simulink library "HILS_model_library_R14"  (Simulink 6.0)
undefined symbols (not defined in the file or in its folder): hilsmdl
libraries: simulink x47, simulink_extras x9, HILS_model_library x3
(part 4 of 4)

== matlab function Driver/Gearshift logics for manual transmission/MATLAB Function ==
function [indicator, skip_nr, req_gear, simtime_prev_out] = fGearVectoMisc(indicator_in, skip_nr_in, last_req_gear, simtime_prev, simtime, act_vehicle_speed, act_rotational_speed,...
                                                            act_gear, clutches_locked, acc_pedal, ref_drive_cycle, gbx, VectoMisc, VectoICE, VectoShiftUp, VectoShiftDown)

% VectoMisc(1,1)    ... dat.vecto.vehicle.mass.value
% VectoMisc(1,2)    ... dat.vecto.fg.ratio.value
% VectoMisc(1,3)    ... dat.vecto.fg.efficiency.value
% VectoMisc(1,4)    ... dat.vecto.wheel.radius.value
% VectoMisc(1,5)    ... dat.vecto.wheel.inertia.value
% VectoMisc(1,6)    ... dat.vecto.wheel.rollingres.value
% VectoMisc(1,7)    ... dat.vecto.aero.af.value
% VectoMisc(1,8)    ... dat.vecto.aero.cd.value
% VectoMisc(1,9)    ... dat.vecto.ICE.idlespeed.value
% VectoMisc(1,10)   ... dat.vecto.ICE.ratedspeed.value
% VectoMisc(1,11)   ... dat.vecto.ICE.starttorquereserve.value
% VectoMisc(1,12)   ... dat.vecto.shiftlocktime.value
% VectoMisc(1,13)   ... dat.clutchtime.value
% VectoMisc(1,14)   ... dat.vecto.skipgears.value
% VectoMisc(1,15)   ... dat.vecto.upshifttorquereserve.value
% VectoMisc(1,16)   ... dat.vecto.startgearengaged.value
% VectoMisc(1,17)   ... dat.vecto.startgearactive.value
                     
% VectoICE(1,:)   ... dat.vecto.ICE.maxtorque_speed.value
% VectoICE(2,:)   ... dat.vecto.ICE.maxtorque_torque.value
% VectoICE(3,:)   ... dat.vecto.ICE.maxtorque_friction.value

% VectoShiftDown(1,:)   ... dat.vecto.downshift_torque.value
% VectoShiftDown(2,:)   ... dat.vecto.downshift_speed.value

% VectoShiftUp(1,:)   ... dat.vecto.upshift_torque.value
% VectoShiftUp(2,:)   ... dat.vecto.upshift_speed.value

% VectoPT1(1,:)   ... dat.vecto.timeconstant_normspeed.value
% VectoPT1(2,:)   ... dat.vecto.timeconstant.value
                        
    persistent lastGearshift;

    %% initialising
    indicator = indicator_in;
    req_gear= last_req_gear;
    simtime_prev_out = simtime_prev;
    skip_nr = 0;
    trq_demand=0;
    n_demand=0;
    n_demand_far_future=0;

    if isempty(lastGearshift)
        lastGearshift = 0;
        indicator = 0;
    end

    maxtorque_speed=VectoICE(1,:);
    maxtorque_torque=VectoICE(2,:);
    maxtorque_friction=VectoICE(3,:);
    downshift_torque=VectoShiftDown(1,:);
    downshift_speed=VectoShiftDown(2,:);
    upshift_torque=VectoShiftUp(1,:);
    upshift_speed=VectoShiftUp(2,:);

    VectoPT1 = zeros(2,11);
    VectoPT1(1,:) = [0 0.538461538 0.615384616 0.692307692 0.769230769 0.846153846 0.923076923 1 1.076923077 1.153846154 10];
    VectoPT1(2,:) = [1 1 0.897471308 0.766055926 0.634640545 0.503225164 0.383742396 0.282872228 0.206491063 0.172580645 0.172580645];
    
    % VectoMisc(1,3)    ... dat.vecto.fg.efficiency.value
        % 'final gear efficiency' [-]
        VectoMisc(1,3) = 0.95;
    % VectoMisc(1,9)    ... dat.vecto.ICE.idlespeed.value
        % 'ICE idle speed' [rad/s]
        VectoMisc(1,9) = min(VectoICE(1,:));
    % VectoMisc(1,11)   ... dat.vecto.ICE.starttorquereserve.value
        % 'minimum ICE torque reserve for start gear detection' [%]
        VectoMisc(1,11) = 30;
    % VectoMisc(1,12)   ... dat.vecto.shiftlocktime.value
        % 'gearchange is suppressed for specified time' [s]
        VectoMisc(1,12) = 3;
    % VectoMisc(1,15)   ... dat.vecto.upshifttorquereserve.value
        % 'minimum ICE torque reserve for skip gears in upshift' [%]
        VectoMisc(1,15) = 30;

       
    

    %% state machine

    switch indicator

        case {0} % standstill

            % start gear will be engaged specified time ("VectoMisc(1,16)=dat.vecto.startgearengaged.value") in advance
            % before the reference cycle value is greater zero
            InterpTime1 = min( (simtime + VectoMisc(1,16)), ref_drive_cycle(end,1) );
            ref_speed_future = interp1( ref_drive_cycle(:,1),ref_drive_cycle(:,2), InterpTime1 );

            req_gear = 0;
            
            % engage start gear for standstill specified time ("VectoMisc(1,16)=dat.vecto.startgearengaged.value") in advance
            InterpTime1 = min( (simtime + VectoMisc(1,16)+5.5), ref_drive_cycle(end,1) );
            if (ref_speed_future > 0 && last_req_gear == 0 && act_vehicle_speed < 0.005 && interp1( ref_drive_cycle(:,1),ref_drive_cycle(:,2), InterpTime1 ) > 0 ) 
                % last condition is to prevent starting in the two small
                % heaps at second 225 and 282 in WHVC cycle
                indicator = 1;
            % engage start gear for slowly rolling vehicle specified time ("VectoMisc(1,16)=dat.vecto.startgearengaged.value") in advance
            elseif (ref_speed_future/VectoMisc(1,4)*VectoMisc(1,2)*gbx(2,2) > (VectoMisc(1,9) + 50*2*pi/60) && last_req_gear == 0 && act_vehicle_speed > 0 && interp1( ref_drive_cycle(:,1),ref_drive_cycle(:,2), InterpTime1 ) > 0 )
                % only shift into start gear "specified clutch time" in
                % advance as soon as cycle reference speed is above idle
                % speed in lowest gear
                indicator = 1;
            end



        case {1} % start

            req_gear=1; % use gear 1 as startgear
            
            if VectoMisc(1,17)==1 % calculate highest possible startgear
                
                % detect highest possible startgear for acceleration with 1.6m/s^2
                % at a vehicle speed of 2m/s
                InterpTime1 = min( (simtime + VectoMisc(1,16)+1), ref_drive_cycle(end,1) );
                trq_demand = (VectoMisc(1,1)+ VectoMisc(1,5)/VectoMisc(1,4)^2)*1.6 + VectoMisc(1,1)*9.81*VectoMisc(1,6) + VectoMisc(1,1)*9.81*sin( interp1( ref_drive_cycle(:,1),ref_drive_cycle(:,3), InterpTime1 ) );       
                trq_demand = trq_demand * VectoMisc(1,4);
                trq_demand = trq_demand / VectoMisc(1,3) / VectoMisc(1,2); % post transmission torque


                for i=2:1:gbx(1,end)
                    pre_trans_trq_demand = trq_demand / gbx(2,i+1) / gbx(3,i+1);
                    n_demand = 2/VectoMisc(1,4) * VectoMisc(1,2) * gbx(2,i+1);  

                    if n_demand < VectoMisc(1,9)
                        break;
                    else
                        %% check if operation point in requested startgear is within shiftig limits
                        % Calculate limits for interpolation from shifting polygones
                        SpeedForReqTorque = min( n_demand, max(maxtorque_speed) );
                        SpeedForReqTorque = max( SpeedForReqTorque, min(maxtorque_speed) );
                        % Calculate limits for interpolation from shifting polygones
                        req_torque = min( pre_trans_trq_demand, interp1( maxtorque_speed, maxtorque_torque,   SpeedForReqTorque ) );
                        req_torque = max( req_torque, interp1( maxtorque_speed, maxtorque_friction, SpeedForReqTorque ) );
                        % Calculate Downshift limit
                        rpmDown = interp1(downshift_torque, downshift_speed, req_torque);
                        if n_demand < rpmDown
                            break;
                        end
                                                
                        act_max_trq   = interp1(maxtorque_speed,   maxtorque_torque,   n_demand);
                    end

                        if (act_max_trq * (100-VectoMisc(1,11))/100) > pre_trans_trq_demand && n_demand > (VectoMisc(1,9) + 100*2*pi/60)
                            
                            InterpTime1 = min( (simtime + VectoMisc(1,16)+5), ref_drive_cycle(end,1) );
                            ref_speed_far_future=interp1( ref_drive_cycle(:,1),ref_drive_cycle(:,2), InterpTime1 ); % 5 sec + specified time ("VectoMisc(1,16)=dat.vecto.startgearengaged.value") in advance
                            n_demand_far_future=ref_speed_far_future/VectoMisc(1,4)*VectoMisc(1,2)*gbx(2,i+1);

                            if n_demand_far_future >= (VectoMisc(1,9) + 200*2*pi/60) % ensures that test cycle ref speed forces at least 200rpm more than idle speed after 5 sec in actual gear (to prevent hight start gear and shift back after short period)
                                req_gear = gbx(1,i+1);
                            end

                        else 
                            break;
                        end
                end
                
            end
            
            indicator = 7;



        case {7} % run in start gear

            req_gear = last_req_gear;

            % Condition for pure electric starting (from 0 rpm to idle speed)
            % if engine speed >= 0.2*normalized engine speed
            if act_rotational_speed >= ( 0.2*(VectoMisc(1,10)-VectoMisc(1,9)) + VectoMisc(1,9)) && clutches_locked == 1 && act_gear == last_req_gear
                indicator = 2;
            end

            % to shift back to N at minicycle 4 and 6, vehicle will never get
            % in run mode there
            InterpTime1 = min( (simtime + VectoMisc(1,16)), ref_drive_cycle(end,1) );
            if (interp1( ref_drive_cycle(:,1),ref_drive_cycle(:,2), InterpTime1 ) == 0)
                indicator = 0;
            end



        case {2} % normal run mode

            % only call case 2 gear determination procedure every 0.2 seconds
            if (simtime-simtime_prev) > 0.2 && (act_gear-floor(act_gear))==0

                simtime_prev_out = simtime;


                %% calculation of shift limits
                % Calculate limits for interpolation from shifting polygones
                SpeedForReqTorque = min( act_rotational_speed, max(maxtorque_speed) );
                SpeedForReqTorque = max( SpeedForReqTorque,    min(maxtorque_speed) );                
                % Calculate max torque demand from actual timestep t until
                % t+shiftlocktime based on reference speed cycle
                trq_demand_max = 0;
                i = simtime;           
                
                while (simtime+VectoMisc(1,12)+0.1) > i
                    % calculate necessary acceleration with
                    % delta speed from [(i+1 second) - i]
                    InterpTime1 = min( (i+1), ref_drive_cycle(end,1) );
                    InterpTime2 = min( i, ref_drive_cycle(end,1) );
                    trq_demand = (VectoMisc(1,1)+ VectoMisc(1,5)/VectoMisc(1,4)^2)*( (interp1(ref_drive_cycle(:,1),ref_drive_cycle(:,2),InterpTime1) - interp1(ref_drive_cycle(:,1),ref_drive_cycle(:,2),InterpTime2) )/(InterpTime1+0.00001-InterpTime2) ) + ...                                  
                                  VectoMisc(1,1)*9.81*VectoMisc(1,6) + VectoMisc(1,1)*9.81*sin( interp1(ref_drive_cycle(:,1),ref_drive_cycle(:,3),InterpTime2) ) + ...                                  
                                  1.2/2*VectoMisc(1,8)*VectoMisc(1,7)*(interp1(ref_drive_cycle(:,1),ref_drive_cycle(:,2),InterpTime2))^2;
                    trq_demand = trq_demand * VectoMisc(1,4);
                    if trq_demand > trq_demand_max
                        trq_demand_max = trq_demand;                        
                    end
                    i = i + 0.5;
                end
                % Calculate max torque demand at actual timestep
                % based on delta (reference speed - actual speed)
                trq_demand = (VectoMisc(1,1)+ VectoMisc(1,5)/VectoMisc(1,4)^2)*( ( interp1(ref_drive_cycle(:,1),ref_drive_cycle(:,2),simtime) - act_vehicle_speed )/1 ) + ...                                  
                                  VectoMisc(1,1)*9.81*VectoMisc(1,6) + VectoMisc(1,1)*9.81*sin( interp1(ref_drive_cycle(:,1),ref_drive_cycle(:,3),simtime) ) + ...                                  
                                  1.2/2*VectoMisc(1,8)*VectoMisc(1,7)*(interp1(ref_drive_cycle(:,1),ref_drive_cycle(:,2),simtime))^2;
                trq_demand = trq_demand * VectoMisc(1,4);
                if trq_demand > trq_demand_max
                    trq_demand_max = trq_demand;                        
                end 
                % Maximum torque is maximum of reference speed based and
                % actual speed based
                trq_demand = trq_demand_max;
                
                % conversion to post transmission torque
                trq_demand = trq_demand / VectoMisc(1,3) / VectoMisc(1,2);
                % conversion to pre transmission torque
                trq_demand = trq_demand / gbx(2,act_gear+1) / gbx(3,act_gear+1);
                % Calculate limits for interpolation from shifting polygones
                req_torque = min( trq_demand, interp1( maxtorque_speed, maxtorque_torque,   SpeedForReqTorque ) );
                req_torque = max( req_torque, interp1( maxtorque_speed, maxtorque_friction, SpeedForReqTorque ) );
                % Calculate Up and Downshift limits
                rpmUp   = interp1(upshift_torque,   upshift_speed,   req_torque);
                rpmDown = interp1(downshift_torque, downshift_speed, req_torque);
               

                %% check for upshift
                if acc_pedal > 0.9
                    
                    if (act_rotational_speed > VectoMisc(1,10)) && (act_gear < gbx(1,end)) && (act_gear == last_req_gear)
                        indicator = 3;
                    end
                    
                else
                    
                    if (act_rotational_speed >= rpmUp) && (act_gear < gbx(1,end)) && (act_gear == last_req_gear)
                        indicator = 3;

                        % check if skip gears is active
                        if (VectoMisc(1,14) == 1) && (act_gear < gbx(1,end-1))

                            % Calculate max torque demand from actual timestep t until
                            % t+shiftlocktime based on reference speed cycle
                            veh_speed_max_torque = 0;
                            trq_demand_max = 0;
                            i = simtime;           

                            while (simtime+VectoMisc(1,12)+0.1) > i
                                % calculate necessary acceleration with
                                % delta speed from [(i+1 second) - i]
                                InterpTime1 = min( (i+1), ref_drive_cycle(end,1) );
                                InterpTime2 = min( i, ref_drive_cycle(end,1) );
                                trq_demand = (VectoMisc(1,1)+ VectoMisc(1,5)/VectoMisc(1,4)^2)*( (interp1(ref_drive_cycle(:,1),ref_drive_cycle(:,2),InterpTime1) - interp1(ref_drive_cycle(:,1),ref_drive_cycle(:,2),InterpTime2) )/(InterpTime1+0.00001-InterpTime2) ) + ...                                  
                                              VectoMisc(1,1)*9.81*VectoMisc(1,6) + VectoMisc(1,1)*9.81*sin( interp1(ref_drive_cycle(:,1),ref_drive_cycle(:,3),InterpTime2) ) + ...                                  
                                              1.2/2*VectoMisc(1,8)*VectoMisc(1,7)*(interp1(ref_drive_cycle(:,1),ref_drive_cycle(:,2),InterpTime2))^2;
                                trq_demand = trq_demand * VectoMisc(1,4);
                                if trq_demand > trq_demand_max
                                    trq_demand_max = trq_demand;  
                                    veh_speed_max_torque = interp1(ref_drive_cycle(:,1),ref_drive_cycle(:,2),InterpTime2);
                                end
                                i = i + 0.2;
                            end
                            % Calculate max torque demand at actual timestep
                            % based on delta (reference speed - actual speed)
                            trq_demand = (VectoMisc(1,1)+ VectoMisc(1,5)/VectoMisc(1,4)^2)*( ( interp1(ref_drive_cycle(:,1),ref_drive_cycle(:,2),simtime) - act_vehicle_speed )/1 ) + ...                                  
                                              VectoMisc(1,1)*9.81*VectoMisc(1,6) + VectoMisc(1,1)*9.81*sin( interp1(ref_drive_cycle(:,1),ref_drive_cycle(:,3),simtime) ) + ...                                  
                                              1.2/2*VectoMisc(1,8)*VectoMisc(1,7)*(interp1(ref_drive_cycle(:,1),ref_drive_cycle(:,2),simtime))^2;
                            trq_demand = trq_demand * VectoMisc(1,4);
                            if trq_demand > trq_demand_max
                                trq_demand_max = trq_demand;
                                veh_speed_max_torque = min(interp1(ref_drive_cycle(:,1),ref_drive_cycle(:,2),simtime),act_vehicle_speed);
                            end 
                            % Calculate post transmission speed and torque
                            % for PT1 (values of actual timestep)
                            post_trans_n_demand_PT1 = min(interp1(ref_drive_cycle(:,1),ref_drive_cycle(:,2),simtime),act_vehicle_speed) / VectoMisc(1,4) * VectoMisc(1,2);
                            % "trq_demand" from line 291 and conversion to post transmission torque
                            trq_demand = trq_demand / VectoMisc(1,3) / VectoMisc(1,2);
                            post_trans_trq_demand_PT1 = trq_demand;
                            
                            % Maximum torque is maximum of reference speed based and
                            % actual speed based
                            trq_demand = trq_demand_max;
                            % conversion to post transmission torque and speed
                            trq_demand = trq_demand / VectoMisc(1,3) / VectoMisc(1,2);
                            post_trans_trq_demand = trq_demand;
                            post_trans_n_demand = veh_speed_max_torque / VectoMisc(1,4) * VectoMisc(1,2);                            

                            % Calculate highest possible gear with enough torque
                            % reserve
                            gear_high = min(gbx(1,end),act_gear+3);
                            for i = (act_gear+2):1:gear_high

                                % Calculate pre transmission speed and torque demand
                                % for new gear
                                pre_trans_n_demand = post_trans_n_demand * gbx(2,i+1);
                                pre_trans_trq_demand = post_trans_trq_demand / gbx(2,i+1) / gbx(3,i+1);
                                pre_trans_n_demand_PT1 = post_trans_n_demand_PT1 * gbx(2,i+1);
                                pre_trans_trq_demand_PT1 = post_trans_trq_demand_PT1 / gbx(2,i+1) / gbx(3,i+1);

                                %% Calculate new shift speed limits for new gear
                                % Calculate limits for interpolation from
                                % shifting polygones for maximum torque value
                                SpeedForReqTorque = min( pre_trans_n_demand, max(maxtorque_speed) );
                                SpeedForReqTorque = max( SpeedForReqTorque,    min(maxtorque_speed) );
                                    % Calculate static max torque
                                    % (for if condition below)
                                    stat_max_trq = interp1(maxtorque_speed,   maxtorque_torque,   SpeedForReqTorque);                                    
                                req_torque = min( pre_trans_trq_demand, interp1( maxtorque_speed, maxtorque_torque,   SpeedForReqTorque ) );
                                req_torque = max( req_torque, interp1( maxtorque_speed, maxtorque_friction, SpeedForReqTorque ) );
                                % Calculate Downshift limits for maximum torque value
                                rpmDown = interp1(downshift_torque, downshift_speed, req_torque);
                                % Calculate limits for interpolation from
                                % shifting polygones for PT1 (actual timestep) torque value
                                SpeedForReqTorque = min( pre_trans_n_demand_PT1, max(maxtorque_speed) );
                                SpeedForReqTorque = max( SpeedForReqTorque,    min(maxtorque_speed) );
                                req_torque = min( pre_trans_trq_demand_PT1, interp1( maxtorque_speed, maxtorque_torque,   SpeedForReqTorque ) );
                                req_torque = max( req_torque, interp1( maxtorque_speed, maxtorque_friction, SpeedForReqTorque ) );
                                % Calculate Downshift limits for PT1 (actual timestep) torque value
                                rpmDown_PT1 = interp1(downshift_torque, downshift_speed, req_torque);

                                %% Calculate actual max torque with new rotational speed
                                % Calculate PT1 time constant for torque buildup
                                timeconstant = interp1(VectoPT1(1,:), VectoPT1(2,:), (SpeedForReqTorque-VectoMisc(1,9))/(VectoMisc(1,10)-VectoMisc(1,9)) );
                                % Calculate dynamic max torque with deltaT = 0.5sec for
                                % PT1 equation like in VECTO
                                act_max_trq = 1/(timeconstant/0.5+1) * ( interp1(maxtorque_speed, maxtorque_torque, SpeedForReqTorque) + timeconstant/0.5*req_torque );

                                %% Check if torque reserve is high enough
                                % Check also if max torque demand from actual timestep t until
                                % t+shiftlocktime can be covered by static fullload
                                % both rotational speeds (maximum torque
                                % and actual timestep) should be above
                                % the respective downshift limit
                                if (act_max_trq * (100-VectoMisc(1,15))/100) > pre_trans_trq_demand_PT1 && pre_trans_n_demand_PT1 > rpmDown_PT1 ...
                                    && pre_trans_n_demand > rpmDown && stat_max_trq >= pre_trans_trq_demand
                                    skip_nr = skip_nr + 1;
                                else
                                    break;
                                end

                            end

                        end

                    end
                    
                end



                %% check for downshift  
              
                if (act_rotational_speed <= rpmDown) && (act_gear > 1) && (act_gear == last_req_gear)
                    indicator = 4;                                        
                elseif (act_rotational_speed < VectoMisc(1,9)) && (act_gear == last_req_gear)
                    indicator = 4;
                end

                req_gear = last_req_gear;

            end



        case {3} % shift up

            req_gear = last_req_gear + 1 + skip_nr_in;
            lastGearshift=simtime;
            indicator = 5;



        case {4} % shift down

            req_gear = last_req_gear - 1 + skip_nr_in;
            lastGearshift=simtime;
            indicator = 6;

                if req_gear==0
                    indicator=0;
                end



        case {5} % upshiftlock

            req_gear = last_req_gear;

            %unlock if
            if ( simtime >= (lastGearshift+VectoMisc(1,12)) && (clutches_locked == 1) ) 
                indicator = 2;
            elseif (act_rotational_speed >= (1.2*(VectoMisc(1,10) - VectoMisc(1,9))+VectoMisc(1,9)) && clutches_locked ==1 ) 
                indicator = 2;
            end



        case {6} % downshiftlock

            req_gear = last_req_gear;

            %unlock if
            if ( simtime >= (lastGearshift+VectoMisc(1,12)) && (clutches_locked == 1) ) 
                indicator = 2;
            elseif ((act_rotational_speed <= (VectoMisc(1,9) + 50*2*pi/60)) && (clutches_locked == 1) && simtime >= (lastGearshift+VectoMisc(1,13)) )
            % it takes some time until the clutch relative speed is high enough
            % and it is detected as open after the driver presses the clutch
            % pedal. the last query ensures that no multiple gearshifts are
            % made when vehicle comes to standstill
                indicator = 2;
            
            % unlock also if clutch is not locked and vehicle speed is zero
            % (i.e. representing braking in neutral gear > after stopping of the vehicle startgear has to be engaged again)
            elseif ( (clutches_locked ~= 1) && act_vehicle_speed < 0.005 )
                req_gear = 0;
                indicator = 0;
            end



        otherwise

            req_gear= last_req_gear;

    % end state machine
    end 


        
% end function
end
